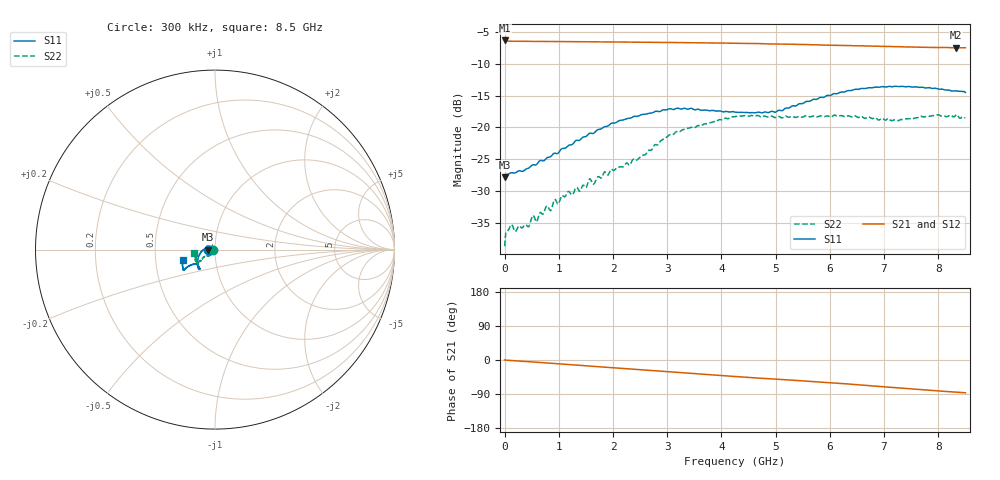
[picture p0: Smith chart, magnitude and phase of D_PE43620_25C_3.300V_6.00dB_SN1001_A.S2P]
! device id: pe43620
! dir: c:\dsa\pe43620\data\pe43620\025c\3p300v\06p00db
! Serial: 1001
! Insertion: A
! Temp: 25C
! VDD: 3.300V
! Attenuation Step: 6.00dB
! IDD: 7.941843e-03mA
! FILE NAME
! DATE 10-22-2008 14:03:43
! CORRECTED  DATA
#  Hz  S  RI  R  50.00
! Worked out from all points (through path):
!   401 points, 300 kHz to 8.5 GHz, reference 50 ohm
!   highest |S21| = -6.37 dB at 300 kHz (marker M1); lowest = -7.5 dB at 8.33 GHz (marker M2)
!   group delay of S21, straight-line fit = 28.1 ps
!   lowest |S11| = -27.8 dB at 300 kHz (marker M3), VSWR 1.08, Z = 46.1 + j0.016 ohm
!   |S11| at or under -10 dB: start of sweep to end of sweep
!   |S22| runs from -38.6 to -18.0 dB; largest |S21 - S12| = 0.0023
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300000  -0.0407 0.000174  0.4803 0.000146  0.4789 0.000398  -0.0117 -0.000239
6.404775e7  -0.0428 6.56e-05  0.474 -0.00631  0.4742 -0.00635  -0.0154 -0.00228
1.065463e8  -0.0439 0.000705  0.4732 -0.0101  0.4739 -0.00994  -0.0167 -0.00267
2.127925e8  -0.0443 0.00253  0.4732 -0.0183  0.4733 -0.0183  -0.015 -0.00364
4.25285e8  -0.0474 0.00482  0.4714 -0.0354  0.4717 -0.0357  -0.0153 -0.00666
5.10282e8  -0.0505 0.00485  0.4704 -0.0424  0.4708 -0.0429  -0.0184 -0.00831
5.95279e8  -0.0512 0.0051  0.4697 -0.0494  0.47 -0.0496  -0.0156 -0.00926
9.35267e8  -0.0627 -0.00188  0.4647 -0.0769  0.4652 -0.0773  -0.02 -0.0185
1.424e9  -0.0806 -0.0168  0.4546 -0.1175  0.4549 -0.1173  -0.0234 -0.0247
1.572745e9  -0.0859 -0.0272  0.4509 -0.1296  0.4511 -0.1295  -0.0257 -0.0303
1.657742e9  -0.0863 -0.0285  0.4483 -0.1364  0.4488 -0.1365  -0.0245 -0.0269
2.125225e9  -0.0963 -0.0598  0.4329 -0.1739  0.4337 -0.1738  -0.0335 -0.0357
2.465213e9  -0.0951 -0.0772  0.4203 -0.2002  0.4206 -0.2006  -0.0439 -0.0358
2.8477e9  -0.0918 -0.0963  0.4044 -0.2276  0.4046 -0.2274  -0.0623 -0.0416
3.315183e9  -0.0891 -0.1096  0.3824 -0.2595  0.3826 -0.2595  -0.0764 -0.0587
4.25015e9  -0.0902 -0.096  0.331 -0.3143  0.3309 -0.3148  -0.0951 -0.0754
4.993874e9  -0.1061 -0.0775  0.2872 -0.3466  0.2862 -0.3469  -0.096 -0.0709
5.67385e9  -0.139 -0.0879  0.2431 -0.3717  0.2435 -0.3725  -0.1048 -0.0628
6.460072e9  -0.1666 -0.1084  0.1865 -0.3948  0.1874 -0.3952  -0.11 -0.0562
7.09755e9  -0.1754 -0.1151  0.1343 -0.4099  0.1339 -0.4098  -0.1075 -0.0435
8.330006e9  -0.1822 -0.0639  0.0379 -0.419  0.0371 -0.4193  -0.1231 -0.0257
8.5e9  -0.1796 -0.0554  0.0259 -0.4205  0.0256 -0.4212  -0.1166 -0.0211
